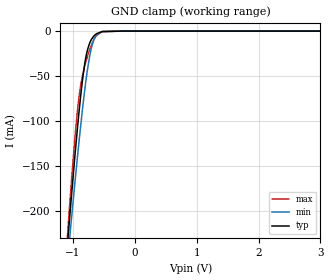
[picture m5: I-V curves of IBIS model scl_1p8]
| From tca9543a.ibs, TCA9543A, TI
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|   scl_1p8 Model
[Model]   scl_1p8
Model_type   Input
Vinl = 0.54
Vinh = 1.26
|   typ   min   max
|   (nom PVT)   (fast PVT)   (slow PVT)
C_comp   3.638e-12   3.557e-12   4.057e-12
[Model spec]
|subparameter
Vinl   0.54   0.504   0.594
Vinh   1.26   1.176   1.386
| Where nom  PVT is Nominal Process, 1.8V, 27C
|   Fast PVT is Strong Process,  1.98V, -40C
|   Slow PVT is Weak Process,   1.68V, 85C
[Voltage Range]   1.8   1.68   1.98
|Junction Temperature
[Temperature Range]   27   85   -40
[Power Clamp Reference]   1.8   1.68   1.98
[GND Clamp Reference]   0   0   0
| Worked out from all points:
|   GND clamp passes 1 mA (typ) near -0.54 V on its own axis
[GND Clamp]
|   Voltage   I(typ)   I(min)   I(max)
-1.8V     -888.9mA   -827.5mA   -994.2mA
-1.095V   -243.7mA   -262.3mA   -235.7mA
-1.058V   -212.8mA   -234.9mA   -200.1mA
-1.022V   -182.7mA   -208.1mA   -166mA
-962.5mV  -135.5mA   -165.6mA   -115.2mA
-914.9mV  -100.1mA   -132.8mA   -81.75mA
-869.4mV  -69.43mA   -102.8mA   -58.66mA
-813.8mV  -39.08mA   -69.01mA   -40.46mA
-761.4mV  -20.43mA   -41.69mA   -27.59mA
-701.3mV  -9.425mA   -18.92mA   -15.76mA
-616mV    -2.86mA    -3.912mA   -4.972mA
3.6V      0A         0A         0A
[POWER Clamp]
|   Voltage   I(typ)   I(min)   I(max)
-1.8V     0A         0A         0A
-1.425V   0A         0A         0A
3.6V      0A         0A         0A
